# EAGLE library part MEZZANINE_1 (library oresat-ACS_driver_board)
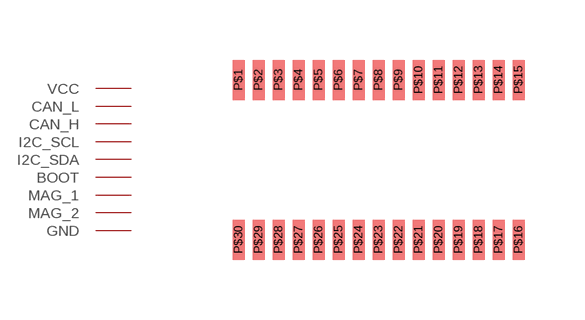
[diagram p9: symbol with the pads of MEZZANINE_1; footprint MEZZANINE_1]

Designator prefix -

## MEZZANINE_1  [MEZZANINE_1]
P$1  GND
P$2  GND
P$3  VCC
P$4  VCC
P$5  CAN_L
P$6  CAN_H
P$7  I2C_SCL
P$8  I2C_SDA
P$9  BOOT
P$10  MAG_1
P$11  MAG_2
P$12  VCC
P$13  VCC
P$14  GND
P$15  GND
P$16  GND
P$17  GND
P$18  VCC
P$19  VCC
P$20  MAG_2
P$21  MAG_1
P$22  BOOT
P$23  I2C_SDA
P$24  I2C_SCL
P$25  CAN_H
P$26  CAN_L
P$27  VCC
P$28  VCC
P$29  GND
P$30  GND

## Footprint MEZZANINE_1 (pad centres in mm)
smd 0.3 x 1: P$1 -3.5,2; P$2 -3,2; P$3 -2.5,2; P$4 -2,2; P$5 -1.5,2; P$6 -1,2; P$7 -0.5,2; P$8 0,2; P$9 0.5,2; P$10 1,2; P$11 1.5,2; P$12 2,2; P$13 2.5,2; P$14 3,2; P$15 3.5,2; P$16 3.5,-2; P$17 3,-2; P$18 2.5,-2; P$19 2,-2; P$20 1.5,-2; P$21 1,-2; P$22 0.5,-2; P$23 0,-2; P$24 -0.5,-2; P$25 -1,-2; P$26 -1.5,-2; P$27 -2,-2; P$28 -2.5,-2; P$29 -3,-2; P$30 -3.5,-2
